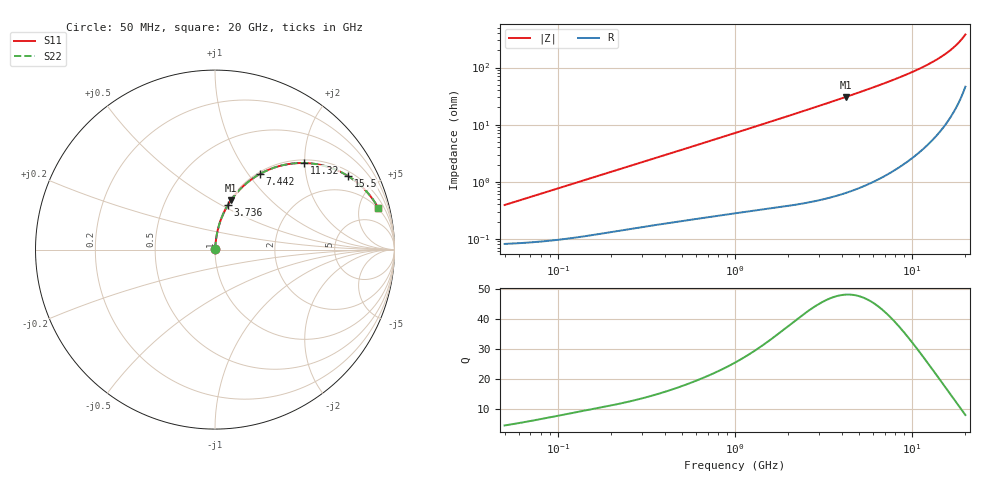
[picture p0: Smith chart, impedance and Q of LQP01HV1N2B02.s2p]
!Murata Part Number: LQP01HV1N2B02
!These Parameters are Measured in Series Mode Connection
!  o--[Z]--o
!Port1  Port2
!  o-------o
!Freq. Start=50[MHz] Stop=20[GHz], 401[Steps]
# Hz S RI R 50
!Freq.(Hz) S11(Real) S11(Imag) S21(Real) S21(Imag) S12(Real) S12(Imag) S22(Real) S22(Imag)
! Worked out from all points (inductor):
!   401 points, 50 MHz to 20 GHz, reference 50 ohm
!   read as one part in series: L = 1.22 nH near 51.52 MHz
!   highest Q = 48 at 4.212 GHz (marker M1), where L = 1.15 nH
!   S11 on the Smith chart (normalised r, x): 50 MHz: 1.00, +0.01; 3.736 GHz: 1.01, +0.54; 7.442 GHz: 1.03, +1.15; 11.32 GHz: 1.07, +1.99; 15.5 GHz: 1.20, +3.50; 20 GHz: 1.93, +7.54
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5e7  0.000828 0.00382  0.9992 -0.00382  0.9992 -0.00382  0.000828 0.00382
1.364002e8  0.00119 0.0103  0.9988 -0.0103  0.9988 -0.0103  0.00119 0.0103
3.721004e8  0.00251 0.027  0.9975 -0.027  0.9975 -0.027  0.00251 0.027
6.380365e8  0.00437 0.0456  0.9956 -0.0456  0.9956 -0.0456  0.00437 0.0456
1e9  0.00781 0.0706  0.9922 -0.0706  0.9922 -0.0706  0.00781 0.0706
1.714689e9  0.0179 0.1191  0.9821 -0.1191  0.9821 -0.1191  0.0179 0.1191
2.728004e9  0.0404 0.1856  0.9596 -0.1856  0.9596 -0.1856  0.0404 0.1856
3.736399e9  0.0718 0.2479  0.9282 -0.2479  0.9282 -0.2479  0.0718 0.2479
4.212059e9  0.0897 0.2755  0.9103 -0.2755  0.9103 -0.2755  0.0897 0.2755
5.683258e9  0.1557 0.3519  0.8443 -0.3519  0.8443 -0.3519  0.1557 0.3519
6.503449e9  0.1987 0.3878  0.8013 -0.3878  0.8013 -0.3878  0.1987 0.3878
7.442007e9  0.2522 0.4222  0.7478 -0.4222  0.7478 -0.4222  0.2522 0.4222
9.178299e9  0.3597 0.4658  0.6403 -0.4658  0.6403 -0.4658  0.3597 0.4658
1.019291e10  0.4253 0.4788  0.5747 -0.4788  0.5747 -0.4788  0.4253 0.4788
1.131968e10  0.4982 0.4825  0.5018 -0.4825  0.5018 -0.4825  0.4982 0.4825
1.334722e10  0.6243 0.4625  0.3757 -0.4625  0.3757 -0.4625  0.6243 0.4625
1.438523e10  0.6838 0.4404  0.3162 -0.4404  0.3162 -0.4404  0.6838 0.4404
1.550395e10  0.7426 0.409  0.2574 -0.409  0.2574 -0.409  0.7426 0.409
1.646126e10  0.7879 0.3769  0.2121 -0.3769  0.2121 -0.3769  0.7879 0.3769
1.747767e10  0.8305 0.3385  0.1695 -0.3385  0.1695 -0.3385  0.8305 0.3385
1.912117e10  0.8869 0.2696  0.1131 -0.2696  0.1131 -0.2696  0.8869 0.2696
2e10  0.9106 0.2305  0.0894 -0.2305  0.0894 -0.2305  0.9106 0.2305
